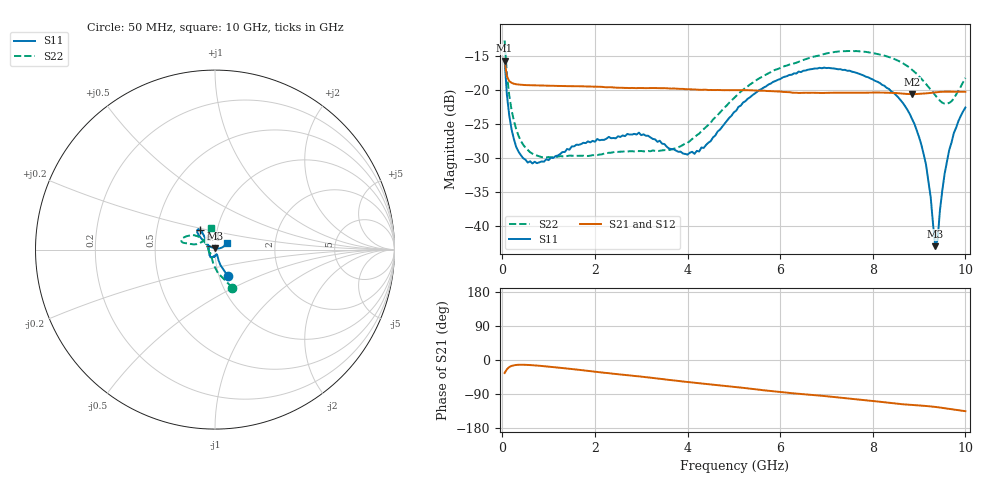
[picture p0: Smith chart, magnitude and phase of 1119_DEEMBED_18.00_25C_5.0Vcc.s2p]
!Hittite Microwave Corp.
!Digital Attenuator/PhaseShifter Rev 1.4.0
!Filename: C:\DATA\DATA\1119_DEEMBED_18.00_25C_5.0Vcc.s2p
!VNA ID: Agilent Technologies,N5224A,MY51441122,A.10.45.03
!Device type:
!2 Port Calibration.
!Temp(C): 25
!Lot Number:
!Serial Number:
!Operator:
!Misc:
!Attenuator:  18.000
# GHZ S DB R 50.0
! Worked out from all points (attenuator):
!   200 points, 50 MHz to 10 GHz, reference 50 ohm
!   highest |S21| = -15.65 dB at 50 MHz (marker M1); lowest = -20.6 dB at 8.85 GHz (marker M2)
!   lowest |S11| = -42.9 dB at 9.35 GHz (marker M3), VSWR 1.01, Z = 49.9 + j0.709 ohm
!   |S11| at or under -10 dB: start of sweep to end of sweep
!   |S22| runs from -29.9 to -12.7 dB; largest |S21 - S12| = 0.00028
!   S11 on the Smith chart (normalised r, x): 50 MHz: 1.10, -0.34; 6.4 GHz: 0.83, +0.18; 10 GHz: 1.14, +0.08
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0.05  -15.58 -64.0  -15.65 -34.4  -15.65 -34.4  -12.68 -65.6
0.1  -20.71 -70.6  -18.00 -24.3  -17.99 -24.3  -17.62 -82.8
0.2  -25.76 -71.0  -18.91 -15.7  -18.91 -15.7  -22.90 -99.6
0.45  -29.99 -67.7  -19.22 -12.5  -19.22 -12.6  -28.00 -120.1
0.85  -30.47 -77.7  -19.31 -15.7  -19.31 -15.8  -29.83 -133.1
1.75  -27.72 -102.6  -19.43 -27.3  -19.43 -27.3  -29.62 -138.5
2.95  -26.23 -120.3  -19.67 -43.2  -19.67 -43.2  -28.95 -157.5
3.4  -27.42 -136.6  -19.69 -49.5  -19.70 -49.5  -28.89 -170.8
4.15  -29.35 177.6  -19.88 -60.1  -19.89 -60.1  -26.93 158.6
5.05  -23.01 133.6  -19.98 -71.4  -20.00 -71.5  -20.84 140.2
6.4  -17.25 127.5  -20.40 -89.0  -20.42 -89.1  -15.82 151.1
6.7  -16.87 129.4  -20.37 -92.3  -20.38 -92.3  -15.10 154.9
7.5  -17.13 135.4  -20.37 -101.8  -20.37 -101.9  -14.23 164.0
8.35  -19.81 140.5  -20.38 -112.8  -20.38 -112.8  -15.12 167.8
8.85  -24.25 144.8  -20.57 -118.6  -20.57 -118.6  -17.00 167.2
9.15  -30.93 147.6  -20.46 -121.3  -20.48 -121.3  -19.08 164.6
9.25  -35.67 140.2  -20.39 -122.5  -20.41 -122.5  -19.91 161.4
9.35  -42.92 96.1  -20.31 -123.8  -20.33 -123.8  -20.74 156.3
9.400001  -41.99 53.8  -20.27 -124.6  -20.29 -124.6  -21.15 152.9
9.5  -34.81 22.1  -20.22 -126.3  -20.24 -126.3  -21.83 143.7
9.65  -28.79 16.1  -20.20 -128.9  -20.21 -128.8  -21.86 126.9
10  -22.54 28.7  -20.22 -135.1  -20.22 -135.0  -18.18 99.6
